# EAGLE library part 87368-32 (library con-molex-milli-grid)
RECEPTACAL
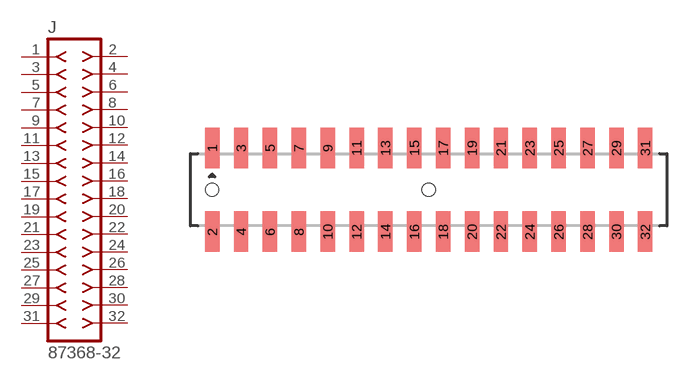
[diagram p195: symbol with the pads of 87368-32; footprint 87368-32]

Designator prefix J

## 87368-32  [87368-32]
1  1  pas
2  2  pas
3  3  pas
4  4  pas
5  5  pas
6  6  pas
7  7  pas
8  8  pas
9  9  pas
10  10  pas
11  11  pas
12  12  pas
13  13  pas
14  14  pas
15  15  pas
16  16  pas
17  17  pas
18  18  pas
19  19  pas
20  20  pas
21  21  pas
22  22  pas
23  23  pas
24  24  pas
25  25  pas
26  26  pas
27  27  pas
28  28  pas
29  29  pas
30  30  pas
31  31  pas
32  32  pas

## Footprint 87368-32 (pad centres in mm)
RECEPTACAL SMD Dual Row, Side Entry
smd 1 x 2.8: 1 -15,2.9; 2 -15,-2.9; 3 -13,2.9; 4 -13,-2.9; 5 -11,2.9; 6 -11,-2.9; 7 -9,2.9; 8 -9,-2.9; 9 -7,2.9; 10 -7,-2.9; 11 -5,2.9; 12 -5,-2.9; 13 -3,2.9; 14 -3,-2.9; 15 -1,2.9; 16 -1,-2.9; 17 1,2.9; 18 1,-2.9; 19 3,2.9; 20 3,-2.9; 21 5,2.9; 22 5,-2.9; 23 7,2.9; 24 7,-2.9; 25 9,2.9; 26 9,-2.9; 27 11,2.9; 28 11,-2.9; 29 13,2.9; 30 13,-2.9; 31 15,2.9; 32 15,-2.9
hole 0.914 at -15,0
hole 0.914 at 0,0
